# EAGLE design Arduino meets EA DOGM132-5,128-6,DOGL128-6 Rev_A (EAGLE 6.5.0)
Assembly variants: DOGM132-5 monochrome, DOGM132-5 RGB, DOGML128 monochrome, DOGML128 RGB
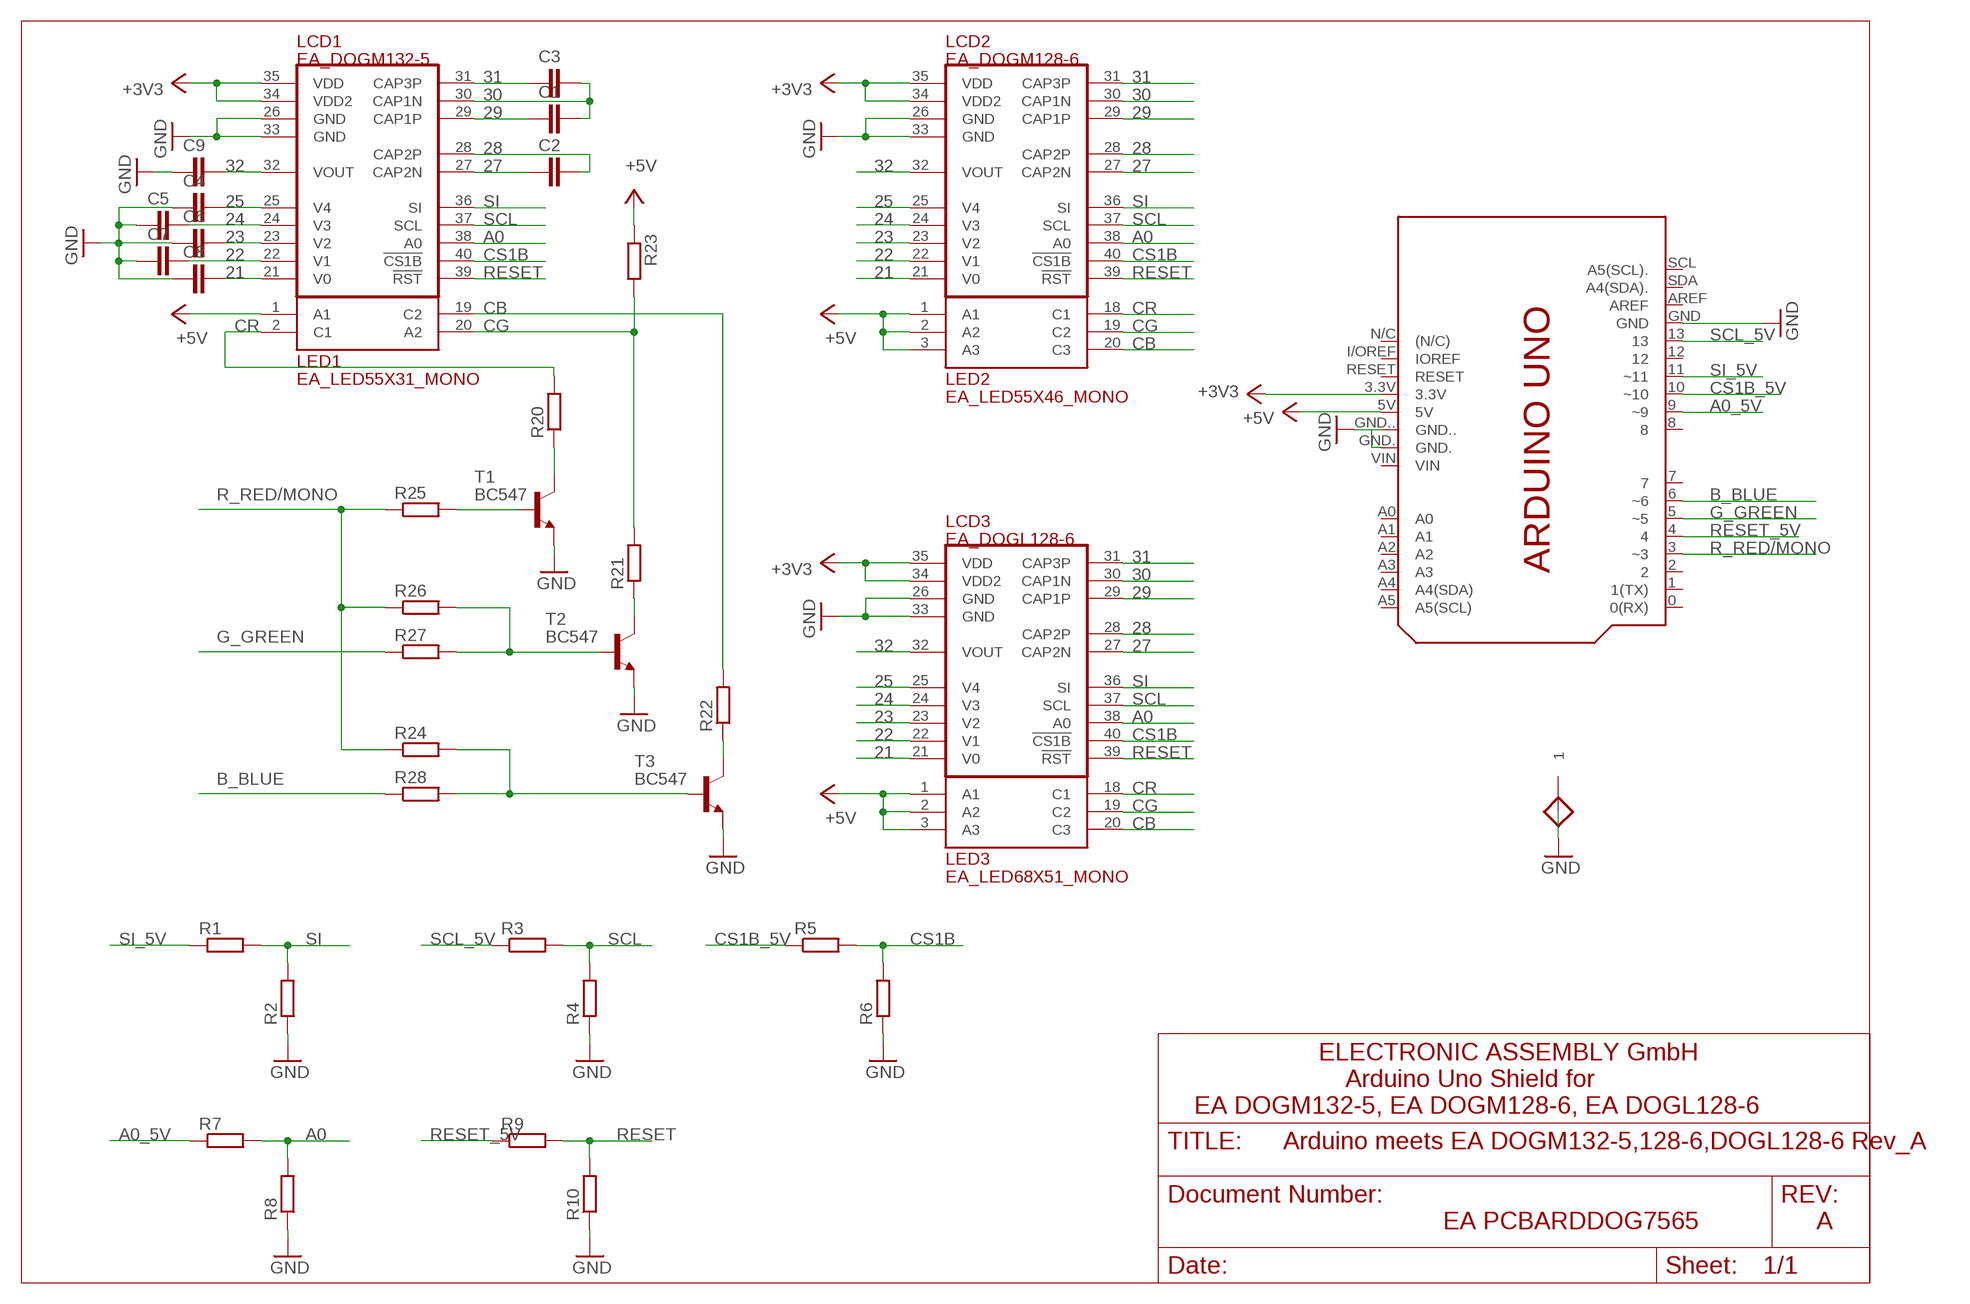
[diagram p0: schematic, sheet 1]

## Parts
C1  1uF  C_5MM_AND_1206  [C_5MM_AND_1206]
C2  1uF  C_5MM_AND_1206  [C_5MM_AND_1206]
C3  1uF  C_5MM_AND_1206  [C_5MM_AND_1206]
C4  1uF  C_5MM_AND_1206  [C_5MM_AND_1206]
C5  1uF  C_5MM_AND_1206  [C_5MM_AND_1206]
C6  1uF  C_5MM_AND_1206  [C_5MM_AND_1206]
C7  1uF  C_5MM_AND_1206  [C_5MM_AND_1206]
C8  1uF  C_5MM_AND_1206  [C_5MM_AND_1206]
C9  1uF  C_5MM_AND_1206  [C_5MM_AND_1206]
GND  PAD55/35  [PAD55/35]
LCD1  EA_DOGM132-5  [EA_DOGM]  (not fitted in variant DOGML128 monochrome)  (not fitted in variant DOGML128 RGB)
LCD2  EA_DOGM128-6  [EA_DOGM128-6]  (not fitted in variant DOGM132-5 monochrome)  (not fitted in variant DOGM132-5 RGB)
LCD3  EA_DOGL128-6  [EA_DOGL128-6]  (not fitted in variant DOGM132-5 monochrome)  (not fitted in variant DOGM132-5 RGB)
LED1  EA_LED55X31_MONO  [EA_LED55X31]  (not fitted in variant DOGML128 monochrome)  (not fitted in variant DOGML128 RGB)
LED2  EA_LED55X46_MONO  [EA_LED55X46]  (not fitted in variant DOGM132-5 monochrome)  (not fitted in variant DOGM132-5 RGB)
LED3  EA_LED68X51_MONO  [EA_LED68X51]  (not fitted in variant DOGM132-5 monochrome)  (not fitted in variant DOGM132-5 RGB)
PCB1  ARDUINO_UNO_SHIELD  [ARDUINO_UNO_SHIELD]
R1  2K7  R_10MM_AND_1206  [R_10MM_AND_1206]
R2  4K7  R_10MM_AND_1206  [R_10MM_AND_1206]
R3  2K7  R_10MM_AND_1206  [R_10MM_AND_1206]
R4  4K7  R_10MM_AND_1206  [R_10MM_AND_1206]
R5  2K7  R_10MM_AND_1206  [R_10MM_AND_1206]
R6  4K7  R_10MM_AND_1206  [R_10MM_AND_1206]
R7  2K7  R_10MM_AND_1206  [R_10MM_AND_1206]
R8  4K7  R_10MM_AND_1206  [R_10MM_AND_1206]
R9  2K7  R_10MM_AND_1206  [R_10MM_AND_1206]
R10  4K7  R_10MM_AND_1206  [R_10MM_AND_1206]
R20  BL_res  R_10MM_AND_1206  [R_10MM_AND_1206]
R21  BL_res  R_10MM_AND_1206  [R_10MM_AND_1206]  (not fitted in variant DOGM132-5 monochrome)
R22  BL_res  R_10MM_AND_1206  [R_10MM_AND_1206]
R23  0R  R_10MM_AND_1206  [R_10MM_AND_1206]  (not fitted in variant DOGM132-5 RGB)  (not fitted in variant DOGML128 monochrome)  (not fitted in variant DOGML128 RGB)
R24  470R  R_10MM_AND_1206  [R_10MM_AND_1206]  (not fitted in variant DOGM132-5 RGB)  (not fitted in variant DOGML128 RGB)
R25  470R  R_10MM_AND_1206  [R_10MM_AND_1206]
R26  470R  R_10MM_AND_1206  [R_10MM_AND_1206]  (not fitted in variant DOGM132-5 monochrome)  (not fitted in variant DOGM132-5 RGB)  (not fitted in variant DOGML128 RGB)
R27  470R  R_10MM_AND_1206  [R_10MM_AND_1206]  (not fitted in variant DOGM132-5 monochrome)  (not fitted in variant DOGML128 monochrome)
R28  470R  R_10MM_AND_1206  [R_10MM_AND_1206]  (not fitted in variant DOGM132-5 monochrome)  (not fitted in variant DOGML128 monochrome)
T1  BC547  [TO92]
T2  BC547  [TO92]  (not fitted in variant DOGM132-5 monochrome)
T3  BC547  [TO92]

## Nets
21: C8.2 LCD1.21(V0) LCD2.21(V0) LCD3.21(V0)
22: C7.2 LCD1.22(V1) LCD2.22(V1) LCD3.22(V1)
23: C6.2 LCD1.23(V2) LCD2.23(V2) LCD3.23(V2)
24: C5.2 LCD1.24(V3) LCD2.24(V3) LCD3.24(V3)
25: C4.2 LCD1.25(V4) LCD2.25(V4) LCD3.25(V4)
27: C2.1 LCD1.27(CAP2N) LCD2.27(CAP2N) LCD3.27(CAP2N)
28: C2.2 LCD1.28(CAP2P) LCD2.28(CAP2P) LCD3.28(CAP2P)
29: C1.1 LCD1.29(CAP1P) LCD2.29(CAP1P) LCD3.29(CAP1P)
30: C1.2 C3.2 LCD1.30(CAP1N) LCD2.30(CAP1N) LCD3.30(CAP1N)
31: C3.1 LCD1.31(CAP3P) LCD2.31(CAP3P) LCD3.31(CAP3P)
32: C9.2 LCD1.32(VOUT) LCD2.32(VOUT) LCD3.32(VOUT)
+3V3: LCD1.34(VDD2) LCD1.35(VDD) LCD2.34(VDD2) LCD2.35(VDD) LCD3.34(VDD2) LCD3.35(VDD) PCB1.3.3V
+5V: LED1.1(A1) LED2.1(A1) LED2.2(A2) LED2.3(A3) LED3.1(A1) LED3.2(A2) LED3.3(A3) PCB1.5V R23.1
A0: LCD1.38(A0) LCD2.38(A0) LCD3.38(A0) R7.2 R8.2
A0_5V: PCB1.9(~9) R7.1
B_BLUE: PCB1.6(~6) R28.1
CB: LED1.19(C2) LED2.20(C3) LED3.20(C3) R22.2
CG: LED1.20(A2) LED2.19(C2) LED3.19(C2) R21.2 R23.2
CR: LED1.2(C1) LED2.18(C1) LED3.18(C1) R20.2
CS1B: LCD1.40(!CS1B!) LCD2.40(!CS1B!) LCD3.40(!CS1B!) R5.2 R6.2
CS1B_5V: PCB1.10(~10) R5.1
G_GREEN: PCB1.5(~5) R27.1
GND: C4.1 C5.1 C6.1 C7.1 C8.1 C9.1 GND.1 LCD1.26(GND) LCD1.33(GND) LCD2.26(GND) LCD2.33(GND) LCD3.26(GND) LCD3.33(GND) PCB1.GND PCB1.GND. PCB1.GND.. R2.1 R4.1 R6.1 R8.1 R10.1 T1.1(E) T2.1(E) T3.1(E)
N$1: R20.1 T1.3(C)
N$2: R21.1 T2.3(C)
N$3: R22.1 T3.3(C)
N$8: R26.2 R27.2 T2.2(B)
N$12: R25.2 T1.2(B)
N$17: R24.2 R28.2 T3.2(B)
R_RED/MONO: PCB1.3(~3) R24.1 R25.1 R26.1
RESET: LCD1.39(!RST!) LCD2.39(!RST!) LCD3.39(!RST!) R9.2 R10.2
RESET_5V: PCB1.4 R9.1
SCL: LCD1.37(SCL) LCD2.37(SCL) LCD3.37(SCL) R3.2 R4.2
SCL_5V: PCB1.13 R3.1
SI: LCD1.36(SI) LCD2.36(SI) LCD3.36(SI) R1.2 R2.2
SI_5V: PCB1.11(~11) R1.1
Unconnected: PCB1.0(0(RX)) PCB1.1(1(TX)) PCB1.2 PCB1.7 PCB1.8 PCB1.12 PCB1.A0 PCB1.A1 PCB1.A2 PCB1.A3 PCB1.A4(A4(SDA)) PCB1.A5(A5(SCL)) PCB1.AREF PCB1.I/OREF(IOREF) PCB1.N/C((N/C)) PCB1.RESET PCB1.SCL(A5(SCL).) PCB1.SDA(A4(SDA).) PCB1.VIN

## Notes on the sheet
- ELECTRONIC ASSEMBLY GmbH
- Arduino Uno Shield for
- EA DOGM132-5, EA DOGM128-6, EA DOGL128-6
- EA PCBARDDOG7565 | A

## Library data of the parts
C1-C9 = EA:C_5MM_AND_1206
GND = EA:PAD55/35
LCD1 = EA:EA_DOGM132-5: ELECTRONIC ASSEMBLY GmbH EA DOGM132B-5 EA DOGM132E-5 EA DOGM132L-5 EA DOGM132S-5 EA DOGM132W-5
LCD2 = EA:EA_DOGM128-6: ELECTRONIC ASSEMBLY GmbH EA DOGM128B-6 EA DOGM128E-6 EA DOGM128L-6 EA DOGM128S-6 EA DOGM128W-6
LCD3 = EA:EA_DOGL128-6: ELECTRONIC ASSEMBLY GmbH EA DOGL128B-6 EA DOGL128E-6 EA DOGL128L-6 EA DOGL128W-6 EA DOGL128S-6
LED1 = EA:EA_LED55X31_MONO
LED2 = EA:EA_LED55X46_MONO: ELECRONIC ASSEMBLY GmbH EA LED55x46-A EA LED55x46-B EA LED55x46-G EA LED55x46-R EA LED55x46-W
LED3 = EA:EA_LED68X51_MONO: ELECRONIC ASSEMBLY GmbH EA LED68x51-A EA LED68x51-B EA LED68x51-G EA LED68x51-R EA LED68x51-W
PCB1 = E14_Arduino:ARDUINO_UNO_SHIELD
R1-R10 R20-R28 = EA:R_10MM_AND_1206
T1-T3 = transistor-npn:BC547: NPN TRANSISTOR

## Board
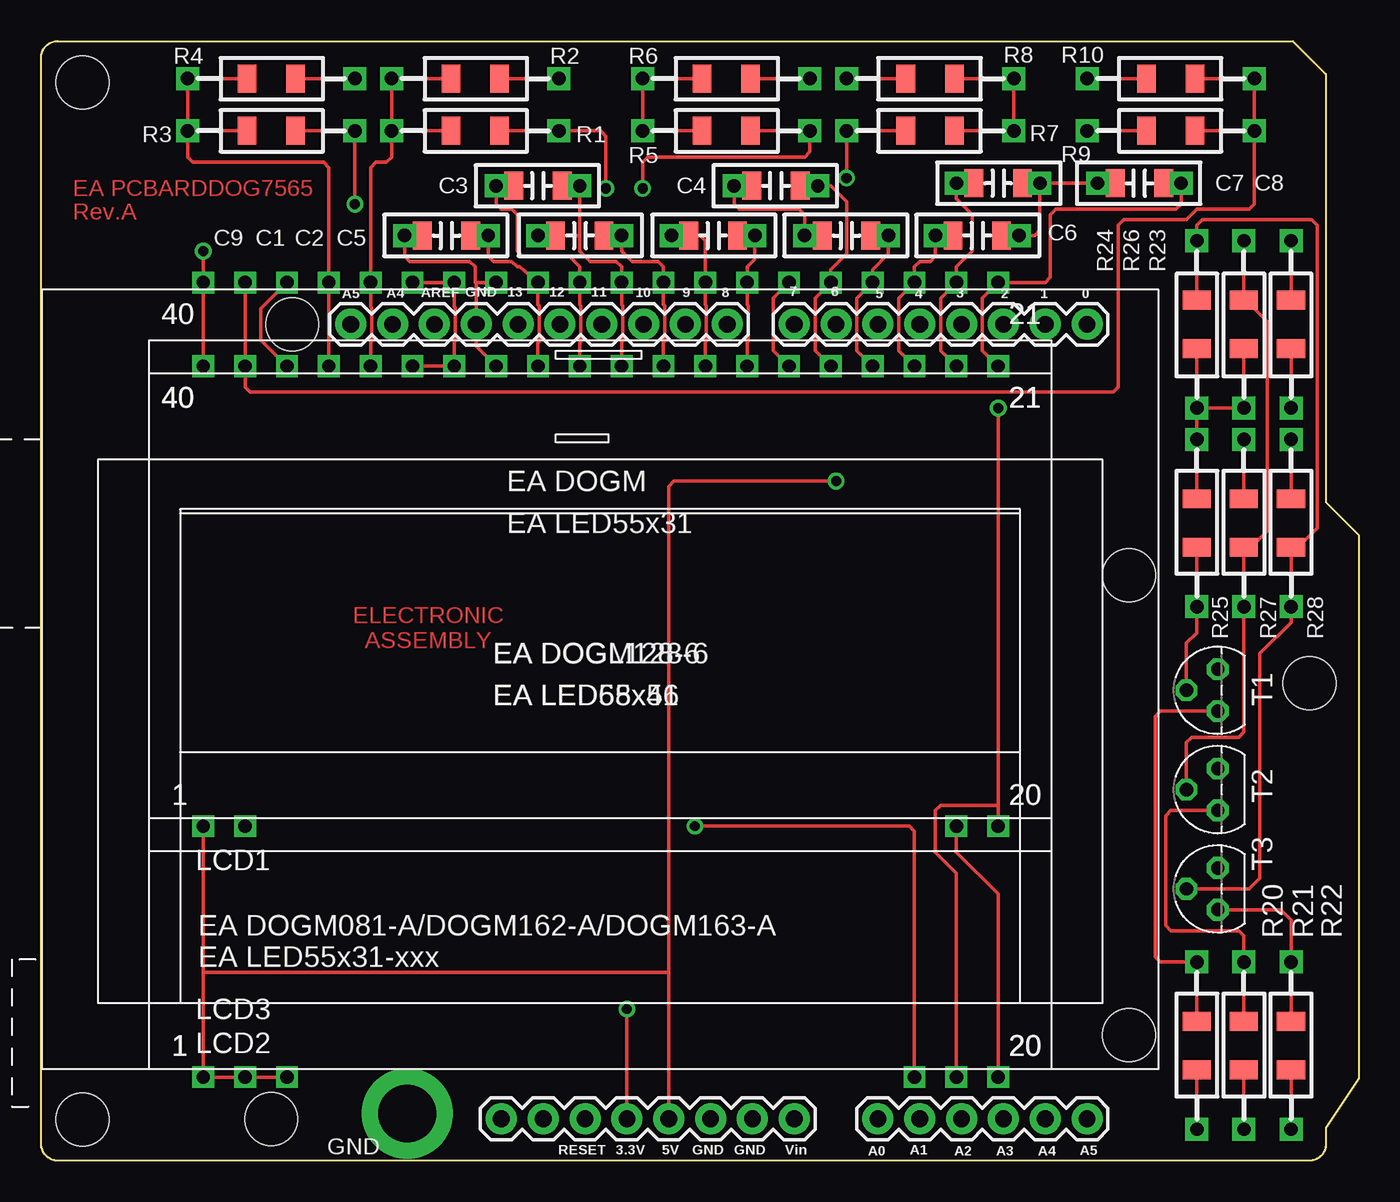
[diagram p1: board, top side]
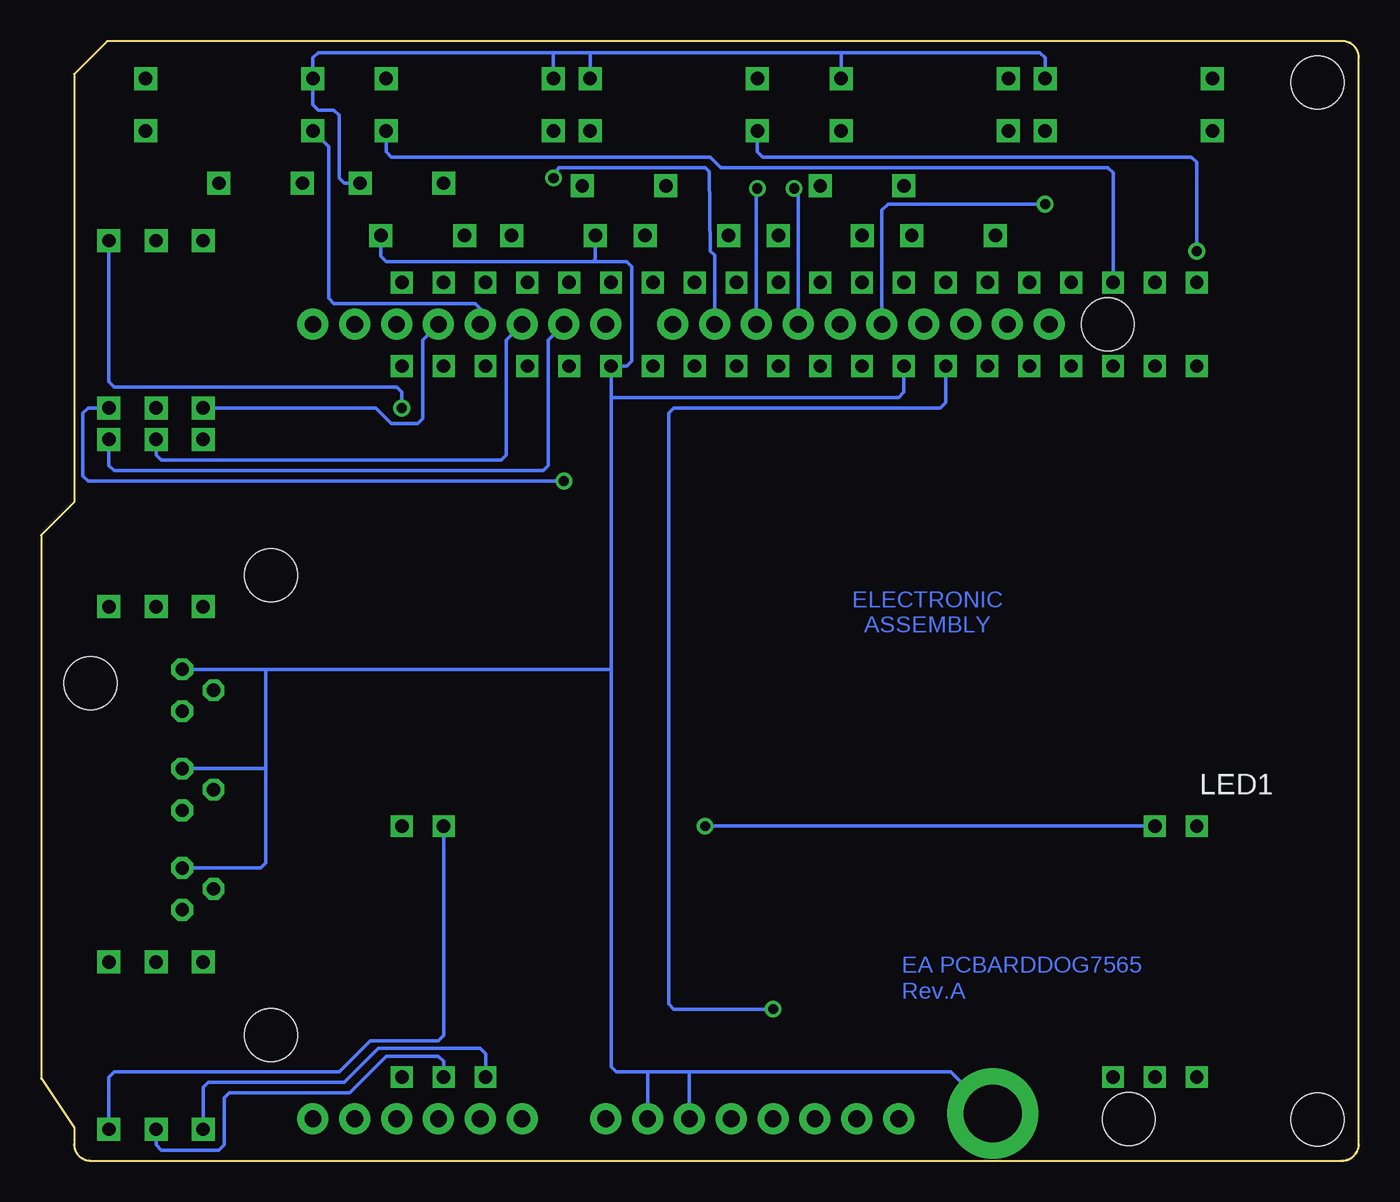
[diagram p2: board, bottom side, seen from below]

Size 80 x 68 mm. Coordinates in mm from the lower left corner, seen from the top.
Outline: 78,2 78,1 arc-90 77,0 1.02,0 arc-90 0,1.02 0,67 arc-90 1,68 76,68 78,66 78,40 80,38 80,5 78,2
Copper layers (1*16): Top 0.035mm / dielectric 1.5mm / Bottom 0.035mm
Design rules "default *": minimum track width 8mil, minimum drill 24mil, track to track 8mil, track to pad 8mil, pad to pad 8mil, via to via 8mil, smd to smd 8mil, copper to edge 40mil, drill to drill 8mil, minimum pad ring 10mil, minimum via ring 8mil, stop-mask expansion 4mil, vias tented up to drill 0mil, thermal gap 10mil
Holes 3.2 mm at 2.5,65.5 2.5,2.5 77,29

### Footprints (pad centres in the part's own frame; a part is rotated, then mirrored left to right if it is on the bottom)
C_5MM_AND_1206 = drill 0.813 pad 1.397 square: 1 0,0; 2 5.08,0 | smd 1.143 x 1.702: 3 4.013,0; 4 1.067,0
PAD55/35 = drill 3.5 pad 5.5: 1 0,0
EA_DOGM = drill 0.813 square: 1 0,0; 2 2.54,0; 19 45.72,0; 20 48.26,0; 21 48.26,27.94; 22 45.72,27.94; 23 43.18,27.94; 24 40.64,27.94; 25 38.1,27.94; 26 35.56,27.94; 27 33.02,27.94; 28 30.48,27.94; 29 27.94,27.94; 30 25.4,27.94; 31 22.86,27.94; 32 20.32,27.94; 33 17.78,27.94; 34 15.24,27.94; 35 12.7,27.94; 36 10.16,27.94; 37 7.62,27.94; 38 5.08,27.94; 39 2.54,27.94; 40 0,27.94
EA_DOGM128-6 = drill 0.813 square: 1 0,0; 2 2.54,0; 3 5.08,0; 18 43.18,0; 19 45.72,0; 20 48.26,0; 21 48.26,43.18; 22 45.72,43.18; 23 43.18,43.18; 24 40.64,43.18; 25 38.1,43.18; 26 35.56,43.18; 27 33.02,43.18; 28 30.48,43.18; 29 27.94,43.18; 30 25.4,43.18; 31 22.86,43.18; 32 20.32,43.18; 33 17.78,43.18; 34 15.24,43.18; 35 12.7,43.18; 36 10.16,43.18; 37 7.62,43.18; 38 5.08,43.18; 39 2.54,43.18; 40 0,43.18
EA_DOGL128-6 = drill 0.813 square: 1 0,0; 2 2.54,0; 3 5.08,0; 18 43.18,0; 19 45.72,0; 20 48.26,0; 21 48.26,48.26; 22 45.72,48.26; 23 43.18,48.26; 24 40.64,48.26; 25 38.1,48.26; 26 35.56,48.26; 27 33.02,48.26; 28 30.48,48.26; 29 27.94,48.26; 30 25.4,48.26; 31 22.86,48.26; 32 20.32,48.26; 33 17.78,48.26; 34 15.24,48.26; 35 12.7,48.26; 36 10.16,48.26; 37 7.62,48.26; 38 5.08,48.26; 39 2.54,48.26; 40 0,48.26
EA_LED55X31 = drill 0.813 square: 1 0,0; 2 2.54,0; 19 45.72,0; 20 48.26,0; 21 48.26,27.94; 22 45.72,27.94; 23 43.18,27.94; 24 40.64,27.94; 25 38.1,27.94; 26 35.56,27.94; 27 33.02,27.94; 28 30.48,27.94; 29 27.94,27.94; 30 25.4,27.94; 31 22.86,27.94; 32 20.32,27.94; 33 17.78,27.94; 34 15.24,27.94; 35 12.7,27.94; 36 10.16,27.94; 37 7.62,27.94; 38 5.08,27.94; 39 2.54,27.94; 40 0,27.94
EA_LED55X46 = drill 0.813 square: 1 0,0; 2 2.54,0; 3 5.08,0; 18 43.18,0; 19 45.72,0; 20 48.26,0; 21 48.26,43.18; 22 45.72,43.18; 23 43.18,43.18; 24 40.64,43.18; 25 38.1,43.18; 26 35.56,43.18; 27 33.02,43.18; 28 30.48,43.18; 29 27.94,43.18; 30 25.4,43.18; 31 22.86,43.18; 32 20.32,43.18; 33 17.78,43.18; 34 15.24,43.18; 35 12.7,43.18; 36 10.16,43.18; 37 7.62,43.18; 38 5.08,43.18; 39 2.54,43.18; 40 0,43.18
EA_LED68X51 = drill 0.813 square: 1 0,0; 2 2.54,0; 3 5.08,0; 18 43.18,0; 19 45.72,0; 20 48.26,0; 21 48.26,48.26; 22 45.72,48.26; 23 43.18,48.26; 24 40.64,48.26; 25 38.1,48.26; 26 35.56,48.26; 27 33.02,48.26; 28 30.48,48.26; 29 27.94,48.26; 30 25.4,48.26; 31 22.86,48.26; 32 20.32,48.26; 33 17.78,48.26; 34 15.24,48.26; 35 12.7,48.26; 36 10.16,48.26; 37 7.62,48.26; 38 5.08,48.26; 39 2.54,48.26; 40 0,48.26
ARDUINO_UNO_SHIELD = drill 1.016 pad 1.88: 0 63.5,50.8; 1 60.96,50.8; 2 58.42,50.8; 3 55.88,50.8; 3.3V 35.56,2.54; 4 53.34,50.8; 5 50.8,50.8; 5V 38.1,2.54; 6 48.26,50.8; 7 45.72,50.8; 8 41.656,50.8; 9 39.116,50.8; 10 36.576,50.8; 11 34.036,50.8; 12 31.496,50.8; 13 28.956,50.8; A0 50.8,2.54; A1 53.34,2.54; A2 55.88,2.54; A3 58.42,2.54; A4 60.96,2.54; A5 63.5,2.54; AREF 23.876,50.8; GND 26.416,50.8; GND. 43.18,2.54; GND.. 40.64,2.54; I/OREF 30.48,2.54; N/C 27.94,2.54; RESET 33.02,2.54; SCL 18.796,50.8; SDA 21.336,50.8; VIN 45.72,2.54 | hole 3.2: 66.04,7.62; 66.04,35.56; 15.24,50.8; 13.97,2.54
R_10MM_AND_1206 = drill 0.813 pad 1.397 square: 1 0,0; 2 10.16,0 | smd 1.143 x 1.702: 3 6.553,0; 4 3.607,0
TO92 = drill 0.813 octagon: 1 1.27,0; 2 0,1.905; 3 -1.27,0

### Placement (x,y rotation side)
C1  35.24,56.2 180 top
C2  43.34,56.2 180 top
C3  27.62,59.21 0 top
C4  42.07,59.21 0 top
C5  46.35,56.2 0 top
C6  59.37,56.2 180 top
C7  60.64,59.37 180 top
C8  64.14,59.37 0 top
C9  22.07,56.2 0 top
GND  22.23,2.86 0 top
LCD1  9.84,20.32 0 top
LCD2  9.84,5.08 0 top
LCD3  9.84,5.08 0 top
LED1  9.84,20.32 0 top
LED2  9.84,5.08 0 top
LED3  9.84,5.08 0 top
PCB1  0,0 0 top
R1  31.43,62.55 180 top
R2  31.43,65.72 180 top
R3  19.05,62.55 180 top
R4  19.05,65.72 180 top
R5  46.67,62.55 180 top
R6  46.67,65.72 180 top
R7  48.9,62.55 0 top
R8  48.9,65.72 0 top
R9  63.5,62.55 0 top
R10  63.5,65.72 0 top
R20  70.17,12.06 270 top
R21  73.03,12.06 270 top
R22  75.88,12.06 270 top
R23  75.88,45.72 90 top
R24  70.17,45.72 90 top
R25  70.17,43.81 270 top
R26  73.03,45.72 90 top
R27  73.03,43.81 270 top
R28  75.88,43.81 270 top
T1  71.44,28.57 90 top
T2  71.44,22.54 90 top
T3  71.44,16.51 90 top

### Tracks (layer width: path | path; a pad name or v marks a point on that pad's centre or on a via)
21
  Top 0.203: LCD2.21 57.15,49.21 57.15,52.39 LCD3.21 60.96,53.34 61.28,53.66 61.28,57.47 61.59,57.78 68.9,57.78 69.22,58.1 C8.2
22
  Top 0.203: LCD2.22 54.61,49.21 54.61,52.39 LCD3.22 55.56,54.29 56.52,55.24 56.52,57.47 55.56,58.42 C7.2
23
  Top 0.203: LCD2.23 52.07,49.21 52.07,52.39 LCD3.23 53.02,54.29 53.34,54.61 53.98,54.61 54.29,54.93 C6.2
24
  Top 0.203: LCD2.24 49.53,49.21 49.53,52.39 LCD3.24 50.48,54.13 51.44,55.09 C5.2
25
  Top 0.203: LCD2.25 46.99,49.21 46.99,52.39 LCD3.25 47.94,54.13 48.9,55.09 48.9,58.26 47.94,59.21 C4.2
27
  Top 0.203: LCD2.27 42.86,49.72 42.93,49.78 42.93,51.94 42.86,52.01 LCD3.27 42.86,54.29 43.34,54.77 C2.1
28
  Top 0.203: LCD2.28 40.32,49.72 40.39,49.78 40.39,51.94 40.32,52.01 LCD3.28 40.32,55.88 40.01,56.2 C2.2
29
  Top 0.203: LCD2.29 37.78,49.72 37.85,49.78 37.85,51.94 37.78,52.01 LCD3.29 37.78,54.29 37.47,54.61 35.88,54.61 35.24,55.24 C1.1
30
  Top 0.203: LCD2.30 35.24,49.72 35.31,49.78 35.31,51.94 35.24,52.01 LCD3.30 35.24,54.29 34.92,54.61 33.34,54.61 32.7,55.24 32.7,56.2 | 32.7,56.2 C1.2 | C3.2 32.7,56.2
31
  Top 0.203: LCD2.31 32.7,49.69 32.77,49.75 32.77,51.94 32.7,52.01 LCD3.31 32.7,54.29 32.07,54.93 29.21,54.93 28.89,55.24 28.89,57.47 28.57,57.78 27.94,57.78 27.62,58.1 C3.1
32
  Top 0.203: C9.2 27.15,54.93 27.46,54.61 28.57,54.61 28.89,54.29 29.05,54.29 LCD3.32 30.16,52.01 30.23,51.94 30.23,49.75 30.16,49.69 LCD1.32
+3V3  (via drill 0.6)
  Top 0.203: LCD3.35 LCD3.34 25.08,51.88 25.15,51.82 25.15,49.78 25.08,49.72 LCD2.34 LCD2.35 | v35.56,9.21 PCB1.3.3V
  Bottom 0.203: LCD2.34 25.08,46.04 25.4,45.72 41.59,45.72 41.91,45.4 41.91,9.53 41.59,9.21 v35.56,9.21
+5V  (via drill 0.61)
  Top 0.203: PCB1.5V 38.1,11.43 | 38.1,11.43 9.84,11.43 | 9.84,11.43 LED1.1 | 9.84,11.43 LED3.1 LED3.2 LED3.3 | 38.1,11.43 38.1,40.96 38.42,41.27 v48.26,41.27
  Bottom 0.203: R23.1 77.15,45.72 77.47,45.4 77.47,41.59 77.15,41.27 v48.26,41.27
A0
  Top 0.203: LCD3.38 13.34,51.75 13.34,49.85 LCD2.38 | R8.2 R7.2
  Bottom 0.203: LCD3.38 14.92,60.01 15.24,60.33 38.73,60.33 39.37,60.96 58.74,60.96 59.05,61.28 R7.2
A0_5V  (via drill 0.61)
  Top 0.203: v48.9,59.69 R7.1
  Bottom 0.203: PCB1.9 39.12,54.99 39.37,55.24 39.43,60.07 39.69,60.33 48.58,60.33 v48.9,59.69
B_BLUE
  Bottom 0.203: R28.1 75.88,42.23 75.56,41.91 49.53,41.91 49.21,42.23 49.21,49.85 PCB1.6
CB
  Top 0.203: LED3.20 58.1,16.19 55.56,18.73 LED1.19
  Bottom 0.203: LED1.19 55.56,7.61 55.88,7.3 60.01,7.3 61.91,5.4 75.56,5.4 75.88,5.08 R22.2
CG  (via drill 0.61)
  Top 0.203: LED3.19 55.56,17.46 54.29,18.73 54.29,21.27 54.61,21.59 58.1,21.59 | 58.1,21.59 LED1.20 | v58.1,45.72 58.1,21.59
  Bottom 0.203: LED3.19 55.56,6.03 55.88,6.35 59.05,6.35 61.28,4.13 68.58,4.13 68.9,3.81 68.9,0.95 69.22,0.64 72.71,0.64 73.03,0.95 R21.2 | v58.1,45.72 58.1,46.67 58.42,46.99 75.56,46.99 75.88,47.31 R23.2
CR  (via drill 0.6)
  Top 0.203: LED3.18 53.02,20 52.7,20.32 v39.69,20.32
  Bottom 0.203: v39.69,20.32 LED1.2 | LED3.18 53.02,6.51 53.34,6.82 59.53,6.82 61.59,4.76 69.85,4.76 70.17,4.45 R20.2
CS1B  (via drill 0.61)
  Top 0.203: LCD2.40 LCD3.40 v9.84,55.24 | R6.2 R5.2
  Bottom 0.203: v9.84,55.24 9.84,60.64 10.16,60.96 36.2,60.96 36.51,61.28 R5.2
CS1B_5V  (via drill 0.61)
  Top 0.203: v36.51,59.05 36.51,60.64 36.83,60.96 46.35,60.96 46.67,61.28 R5.1
  Bottom 0.203: PCB1.10 36.58,58.99 v36.51,59.05
G_GREEN
  Bottom 0.203: R27.1 73.03,42.86 72.71,42.55 52.07,42.55 51.75,42.86 51.75,49.85 PCB1.5
GND
  Top 0.203: LCD3.26 44.45,52.39 44.45,49.21 LCD2.26 | LCD2.33 26.42,49.47 PCB1.GND 26.42,53.28 26.35,53.34 | C6.1 60.33,56.2 60.64,56.52 C7.1 C8.1 | C5.1 46.35,57.47 46.04,57.78 42.39,57.78 42.07,58.1 C4.1 | C9.1 22.07,54.93 22.38,54.61 26.04,54.61 26.35,54.29 26.35,53.34 | 26.35,53.34 LCD3.33
  Bottom 0.203: PCB1.GND. 43.18,5.4 | 43.18,5.4 40.64,5.4 | 40.64,5.4 PCB1.GND.. | GND.1 24.77,5.4 40.64,5.4 | 43.18,5.4 45.09,5.4 45.4,5.71 45.4,29.84 | 45.4,29.84 66.36,29.84 | 66.36,29.84 T1.1 | T2.1 66.36,23.81 | 66.36,23.81 66.36,29.84 | T3.1 66.67,17.78 66.36,18.1 66.36,23.81 | 45.4,46.35 LCD2.26 44.45,48.26 44.13,48.58 44.13,54.29 44.45,54.61 46.51,54.61 | 45.4,46.35 45.4,29.84 | 45.4,46.35 27.94,46.35 27.62,46.67 LCD2.33 | C6.1 59.37,54.93 59.05,54.61 46.51,54.61 | C5.1 46.35,54.77 46.51,54.61 | R4.1 19.05,66.99 19.37,67.31 31.43,67.31 | 31.43,67.31 R2.1 | R6.1 46.67,67.31 | 46.67,67.31 31.43,67.31 | R8.1 48.9,67.31 | 48.9,67.31 46.67,67.31 | 48.9,67.31 63.18,67.31 63.5,66.99 R10.1 63.5,64.14 63.18,63.82 62.23,63.82 61.91,63.5 61.91,59.69 61.59,59.37 C7.1
N$1
  Top 0.203: T1.3 67.94,27.3 67.63,26.99 67.63,12.38 67.94,12.06 R20.1
N$2
  Top 0.203: T2.3 68.58,21.27 68.26,20.95 68.26,14.29 68.58,13.97 72.71,13.97 73.03,13.65 R21.1
N$3
  Top 0.203: T3.3 75.25,15.24 75.88,14.61 R22.1
N$8
  Top 0.203: 73.03,36.83 74.45,38.26 74.45,50.96 73.03,52.39 73.03,52.7 | T2.2 69.53,25.4 69.85,25.72 72.71,25.72 73.03,26.04 R27.2
N$12
  Top 0.203: T1.2 69.53,31.43 70.17,32.07 R25.2
N$17
  Top 0.203: 75.88,36.83 77.47,38.42 77.47,56.83 77.15,57.15 70.48,57.15 70.17,56.83 R24.2 | T3.2 73.34,16.51 73.98,17.14 73.98,30.8 75.88,32.7 R28.2
R_RED/MONO
  Top 0.203: R25.1 R24.1 R26.1
  Bottom 0.203: PCB1.3 56.83,49.85 56.83,45.09 57.15,44.77 58.74,44.77 59.69,45.72 R24.1
RESET
  Top 0.203: LCD3.39 LCD2.39 12.38,46.99 12.7,46.67 65.09,46.67 65.41,46.99 65.41,56.83 65.72,57.15 69.53,57.15 70.17,57.78 73.34,57.78 73.66,58.1 R9.2 R10.2
RESET_5V
  Bottom 0.203: PCB1.4 53.34,51.75 53.66,52.07 62.23,52.07 62.55,52.39 62.55,61.59 R9.1
SCL
  Top 0.203: LCD2.37 LCD3.37 17.46,60.33 17.14,60.64 9.21,60.64 8.89,60.96 R3.2 R4.2
SCL_5V  (via drill 0.61)
  Top 0.203: v19.05,58.1 R3.1
  Bottom 0.203: PCB1.13 28.96,57.72 28.57,58.1 v19.05,58.1
SI
  Top 0.203: LCD2.36 20,49.72 20.07,49.78 20.07,51.81 20,51.87 LCD3.36 20,60.33 20.32,60.64 20.95,60.64 21.27,60.96 R1.2 R2.2
SI_5V  (via drill 0.61)
  Top 0.203: v34.29,59.05 34.29,62.23 33.97,62.55 R1.1
  Bottom 0.203: PCB1.11 34.04,58.8 v34.29,59.05

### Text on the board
Top: EA PCBARDDOG7565 | Rev.A | ELECTRONIC / ASSEMBLY
Bottom: ELECTRONIC / ASSEMBLY | EA PCBARDDOG7565 | Rev.A
tPlace: EA DOGM081-A/DOGM162-A/DOGM163-A | EA LED55x31-xxx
